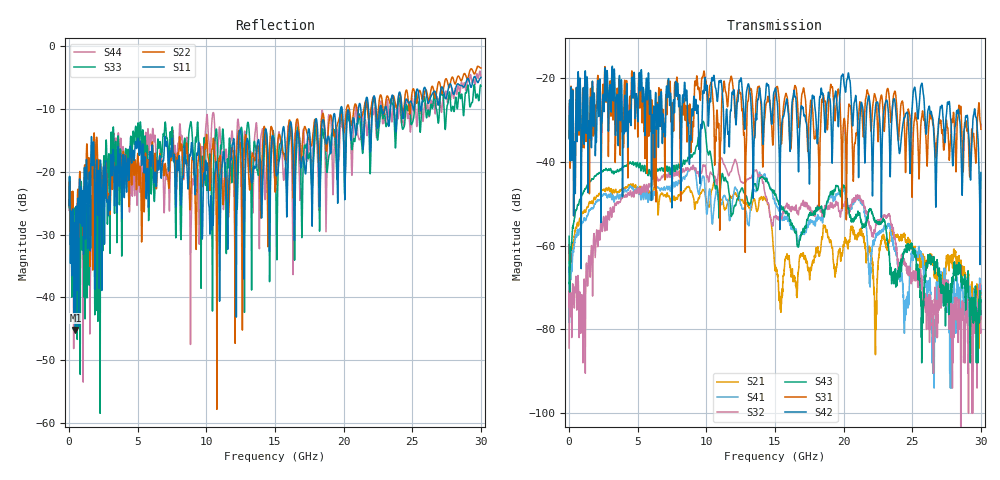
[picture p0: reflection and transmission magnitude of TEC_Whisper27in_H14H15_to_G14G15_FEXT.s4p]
! Tyco Electronics
! H14H15-G14G15_FEXT
!! PART DESCRIPTION: Whisper 27in Megtron 6 VLP-HVLP-VLP Channel Model, bulkhead 2.4mm test pts
!! MODEL DESCRIPTION: System 4-port S-parameter
!! MODEL STATUS: Measured
!! MODEL GEOMETRY: Channel Model
!! MODEL FREQUENCY RANGE: DC to 30.000 GHz in 10.000 MHz frequency steps
!! MODEL EDGE RATE LIMITATION: 12.500 ps (Using conservative 0.5/Fmax rule of thumb)
!! TIME-DOMAIN TRANSFORM CAUTIONS:
!! 1.) Do not simulate transient edge rates faster than the number listed above.  Edge rates faster than this number
!!  contain significant spectral content at frequencies above the model's highest frequency.
!! 2.) Even when simulating edge rates that are slower than the number listed above, be aware that the best time
!!  resolution possible with a direct iFFT is (1 / 2Fmax).  As a result, time resolution is typically not adequate
!!  for most time-domain simulations unless tricks such as windowing are used to minimize leakage and aliasing.
!! 3.) Because the model has a uniform frequency step, a direct iFFT will result in an impulse that that has a time
!!  length given by either (1 / Fstep) or (1 / 2Fstep), depending on the transform being used.  Care has been taken
!!  in selecting the frequency step to ensure a settled impulse response for the model.  Therefore, convolution with
!!  the model's impulse response should present no issues.  However, if directly concatenating s-parameter models
!!  in the frequency domain a user must either interpolate necessary interim frequencies or complete impulse response
!!  zero-padding.  Impulse response zero-padding is more difficult, but more accurate.
!! PORT DEFINITIONS:
!! Port  1  ----->  Side A  H14  G14  Side B  <-----  Port  2
!! Port  3  ----->  Side A  H15  G15  Side B  <-----  Port  4
! Point-to-Point link (differential)  !
! Connectors:  !
!  1: STRADA Whisper  !
! Materials:  !
!  Backplane: Megtron-6 HVLP  !
!  Daughtercard: Megtron-6 VLP  !
! Stack-up:  !
!  Backplane: 20 layers, 200mil thick  !
!  Daughtercard: 14 layers, 110mil thick  !
! Trace Length:  !
!  Backplane: 17in  !
!  Daightercards: 5in  !
! Trace Width:  !
!  Backplane: 8-13-8 mils  !
!  Daughtercards: 6-9-6 mils  !
! Geometry:  !
!  Backplane: Stripline  !
!  Daughtercards: Stripline  !
! Freq. Range: 0 GHz - 30 GHz  !
! Note1: non-mixed-mode s-parameters  !
! Note2: channel includes 2.4mm test points  !
! Touchstone data converted from IdEM dataset
# GHz S MA R 50
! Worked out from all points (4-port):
!   3000 points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, 10 MHz to 30 GHz, reference 50 ohm
!   strongest paths, dB at 10 MHz, 7.51 GHz, 15.01 GHz, 22.51 GHz, 30 GHz:
!     S42: -34.5, -40.8, -22.7, -26.3, -42.6
!     S31: -34.2, -26.1, -24.4, -35.2, -32.3
!     S43: -57.8, -42.1, -47.9, -54.6, -76.5
!     S32: -84.4, -44.2, -53.3, -54.0, -80.0
!     S41: -66.7, -46.3, -50.1, -56.8, -71.7
!     S21: -59.7, -49.0, -66.0, -64.6, -71.4
!   lowest |S11| = -45.2 dB at 470 MHz (marker M1), VSWR 1.01, Z = 50.5 + j0.253 ohm
!   |S11| at or under -10 dB: start of sweep to 19.79 GHz; 19.9 GHz to 21.08 GHz (1.184 GHz wide, 5.78 % of centre); 21.25 GHz to 21.56 GHz (309.3 MHz wide, 1.44 % of centre)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
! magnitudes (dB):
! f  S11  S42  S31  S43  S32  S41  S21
! 10 MHz  -25.3  -34.5  -34.2  -57.8  -84.4  -66.7  -59.7
! 470 MHz  -45.2  -41.1  -40.5  -52.0  -70.2  -57.7  -55.9
! 11.09 GHz  -21.1  -20.8  -30.8  -44.3  -39.1  -50.2  -49.1
! 14.32 GHz  -13.1  -24.2  -27.0  -44.6  -48.3  -44.1  -49.1
! 15.41 GHz  -16.8  -37.2  -32.8  -50.9  -54.0  -52.7  -75.4
! 25.7 GHz  -9.2  -21.3  -29.2  -84.4  -68.4  -62.4  -64.3
! 30 GHz  -5.0  -42.6  -32.3  -76.5  -80.0  -71.7  -71.4
